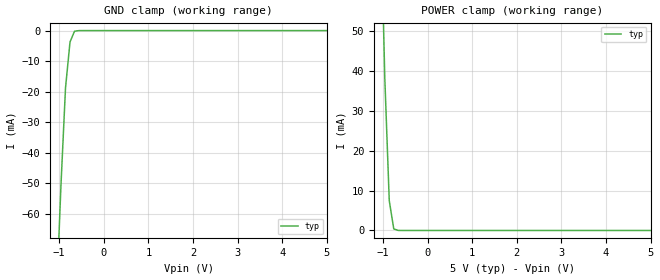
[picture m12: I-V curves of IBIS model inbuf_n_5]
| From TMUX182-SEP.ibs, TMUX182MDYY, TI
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| inbuf_n_5
[Model]   inbuf_n_5
Model_type   Input
Vinl = 0.8
Vinh = 1.35
|   typ   min   max
C_comp   6.362683e-13   NA   NA
[Voltage Range]   5   NA   NA
[Temperature Range]   27   NA   NA
[Power Clamp Reference]   5   NA   NA
[GND Clamp Reference]   0   NA   NA
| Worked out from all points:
|   GND clamp passes 1 mA (typ) near -0.68 V on its own axis
|   POWER clamp passes 1 mA (typ) near -0.77 V on its own axis
[GND Clamp]
|   Voltage   I(typ)   I(min)   I(max)
-5V       -2.674A    NA         NA
-1.061V   -87.09mA   NA         NA
-959.6mV  -50.28mA   NA         NA
-858.6mV  -18.75mA   NA         NA
-757.6mV  -3.722mA   NA         NA
-656.6mV  -214.7uA   NA         NA
-454.5mV  -1.233uA   NA         NA
5V        66.3nA     NA         NA
[POWER Clamp]
|   Voltage   I(typ)   I(min)   I(max)
-5V       3.151A     NA         NA
-1.061V   85.92mA    NA         NA
-959.6mV  38.53mA    NA         NA
-858.6mV  7.471mA    NA         NA
-757.6mV  393.6uA    NA         NA
-656.6mV  10.22uA    NA         NA
-555.6mV  305.2nA    NA         NA
5V        -416.3nA   NA         NA
